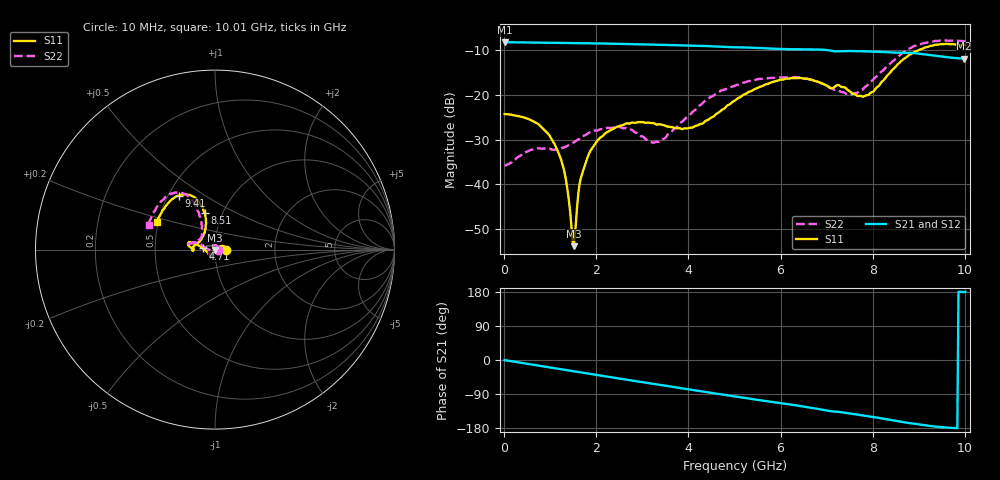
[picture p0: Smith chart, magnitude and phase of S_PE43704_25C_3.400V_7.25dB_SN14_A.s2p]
! Device ID: PE43704
! Dir: z:\PE43704\PE43704_Char_1_20130516\PE43704\AMB\3p400V\7p25dB
! Serial: 14
! Insertion: A
! Impedance: 50 ohm
! Temp: Amb
! VDD: 3.400V
! Attenuation Step: 7.25dB
! IDD: 1.140316e-01mA
#  Hz  S  RI  R  50
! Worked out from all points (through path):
!   401 points, 10 MHz to 10.01 GHz, reference 50 ohm
!   highest |S21| = -8.27 dB at 10 MHz (marker M1); lowest = -11.9 dB at 9.985 GHz (marker M2)
!   group delay of S21, straight-line fit = 51.5 ps
!   lowest |S11| = -53.8 dB at 1.51 GHz (marker M3), VSWR 1.00, Z = 50.1 - j0.172 ohm
!   |S11| at or under -10 dB: start of sweep to 9.004 GHz
!   |S22| runs from -35.9 to -7.9 dB; largest |S21 - S12| = 0.0028
!   S11 on the Smith chart (normalised r, x): 10 MHz: 1.13, +0.00; 4.71 GHz: 0.88, +0.01; 8.51 GHz: 0.83, +0.35; 9.41 GHz: 0.57, +0.39; 10.01 GHz: 0.49, +0.17
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1e7  0.0608 0.000203  0.3861 -0.00158  0.3862 -0.00136  0.016 0.000431
6.85e8  0.0446 0.02  0.3714 -0.0903  0.3714 -0.0901  0.00445 0.0245
1.06e9  0.0253 0.0161  0.3555 -0.1361  0.3555 -0.1359  -0.0111 0.0215
1.285e9  0.0129 0.00846  0.3425 -0.1625  0.3425 -0.1624  -0.0213 0.0145
1.46e9  0.00336 0.00025  0.3313 -0.1819  0.3314 -0.1817  -0.0275 0.00695
1.51e9  0.00111 -0.00172  0.3278 -0.1874  0.328 -0.1872  -0.029 0.00468
1.685e9  -0.00728 -0.0104  0.3153 -0.206  0.3153 -0.2058  -0.0339 -0.00369
1.885e9  -0.0146 -0.0194  0.2994 -0.2258  0.2995 -0.2256  -0.0359 -0.0124
2.235e9  -0.0211 -0.032  0.2686 -0.2575  0.2688 -0.2574  -0.0371 -0.0213
3.36e9  -0.0251 -0.0393  0.1512 -0.3277  0.1516 -0.3274  -0.0287 -0.00794
4.035e9  -0.0379 -0.0198  0.0732 -0.3454  0.0737 -0.3455  -0.0583 0.0141
4.71e9  -0.0665 0.00645  -0.0047 -0.3437  -0.00455 -0.3434  -0.1044 0.039
5.01e9  -0.0842 0.019  -0.0365 -0.3372  -0.036 -0.3373  -0.1217 0.0348
5.935e9  -0.1374 0.0417  -0.1251 -0.2994  -0.1243 -0.3003  -0.1514 0.0339
6.685e9  -0.1452 0.0195  -0.1907 -0.2576  -0.1907 -0.2574  -0.1418 0.0343
7.585e9  -0.0952 0.0372  -0.244 -0.1863  -0.2435 -0.186  -0.0781 0.0687
7.91e9  -0.0663 0.0745  -0.2591 -0.1581  -0.2599 -0.1596  -0.0711 0.1108
8.36e9  -0.0507 0.1654  -0.2746 -0.1137  -0.2743 -0.1148  -0.0881 0.199
8.51e9  -0.0557 0.2019  -0.2785 -0.0968  -0.2777 -0.0983  -0.1017 0.2349
9.41e9  -0.2018 0.3003  -0.2697 -0.0178  -0.2697 -0.0167  -0.2616 0.3001
9.985e9  -0.3189 0.1626  -0.2533 0.00216  -0.254 0.00328  -0.3657 0.1462
1.001e10  -0.3245 0.1524  -0.2541 0.00232  -0.2552 0.00245  -0.3691 0.1376
